FUNCTION_BLOCK FB_SFP_PPD_IO_LINK_ACYCLIC_DATA_V1_0_0
//-------------------------------------
VAR_INPUT

b_RELEASE								: BOOL;
i_READ_WRITE							: INT; 						// 1 = Read Index / 2 = Read All Parameter / 3 = Wright Index / 4 = Wright All Parameter
b_START									: BOOL;
s_NETID 								: STRING(23); 				// T_AmsNetId
i_IO_LINK_PORT_NR						: UINT;						// Port Number of IO-Link Master
w_INDEX 								: WORD			:= 16#00;
i_AREA_A								: INT;						// Parameter 66
i_AREA_B								: INT;						// Parameter 67
di_PISTON_STROKE : DINT;											// Parameter 68
di_FINGER_STROKE						: DINT;						// Parameter 177
ui_PREPOSITION_DELTA					: UINT;						// Parameter 178

END_VAR
//-------------------------------------
VAR_OUTPUT
	
    b_DONE											: BOOL;
    b_BUSY 											: BOOL;
    b_ERROR 										: BOOL;
	i_AREA_A_READ									: INT;	// Parameter 16#66
	i_AREA_B_READ									: INT;	// Parameter 16#67
	di_PISTON_STROKE_READ 	: DINT;	// Parameter 16#68
	di_FINGER_STROKE_READ							: DINT; // Parameter 16#177
	ui_PREPOSITION_DELTA_READ						: UINT; // Parameter 16#178

END_VAR
//-------------------------------------
VAR_STAT
	// Ab Hier soll alles Stat_Var sein
	
	Read_Write_Started	: BOOL; // Hilfsbit welches sich merkt, dass das Lesen und schreiben schon mal angestoßen wurde
	Index				: WORD;	// Index welcher über die Eingangsdaten eingelesen wird wird hier gespeichert
	Next_Parameter		: INT; // Welcher Parameter soll gelesen/geschrieben werden
	Next_Parameter_OLD	: INT; // Welcher Parameter wurde gelesen/geschrieben
	
// Struktur der Aktuell eingelesenen Parameter
	Parameter_Aktuell_i_Area_A									: INT; // 0x66 
	Parameter_Aktuell_i_Area_B									: INT; // 0x67
	Parameter_Aktuell_di_PISTON_STROKE	: DINT; // 0x68
	Parameter_Aktuell_di_Finger_Stroke							: DINT; // 0x177
	Parameter_Aktuell_di_Preposition_Delta						: UINT; // 0x178
	
	// Flanke zur Auswertung des Start Eingangs
	R_TRIG_instance_START	: R_TRIG;
	R_TRIG_instance_START_Q : BOOL;
	
	R_TRIG_WRREC_Error		: R_TRIG; // Triggerauswertung wenn beim Schreiben von Parametern etwas schiefgegangen ist
	R_TRIG_WRREC_Error_Q	: BOOL;
	
	
	Count_Write 		: INT; // Interner Hilfszähler
	Count_Write_Error 	: INT; // Interner schreib Fehlerzähler
	
	help_Valid_Done 	: BOOL; // Hilfsbit das Lesen oder Schreiben fertig sind
	help_Error 			: BOOL; // Hilfsbit Wenn ein Fehler auftritt

	// Struktur um Interne Error Bits auszuwerten 
	Error_struct_Error_Read_Write						: BOOL;
	Error_struct_Area_A									: BOOL;
	Error_struct_Area_B									: BOOL;
	Error_struct_PISTON_STROKE	: BOOL;
	Error_struct_Finger_Stroke							: BOOL;
	Error_struct_Preposition_Delta						: BOOL;
	
	Help_Index_Counter 									: DINT; // Bei Schritt 99 wird der letzte Index gesichert
		
	// Bausteine aus IO_Link Lib
	FB_IolRead				: FB_IolRead;
	FB_IolWrite				: FB_IolWrite;
		
	// Funktionsbausteine 
	FB_Parameter_Lesen_ADSREAD 		: ADSREAD;	// Funktionsbaustein zum Daten Azyklisch lesen 
	FB_Parameter_Schreiben_ADSWRITE	: ADSWRITE; // Funktionsbaustein zum Daten Azyklisch schreinen

	
	dw_Help_Storage_Copy	: DWORD;
	uint_Help_Storage_Copy	: UINT;
	dw_Help_Storage_Write	: DWORD;
	b_Help_Busy				: BOOL;
	
	// Zeit
	//FB_Time_Delay_Valid_Done : ton;

	t_Timeout : TIME := DEFAULT_ADS_TIMEOUT;
	 
	// ADSREAD Varriablen
	// OUTPUT	  
	  
	Length_DATA_WRITE	: UDINT;

	// Read Parameter 
		
	Help_last_round: BOOL;
	
	Help_Wartezeit: TON;
	Help_Wartezeit_Q : BOOL;
	Help_Wartezeit_time: TIME;
	
	Test_B_Trig_Start_Q: BOOL;
	temp_FB_IolWrite_bDone_Help: BOOL;
END_VAR	

//#################	
VAR	

END_VAR	  

//#################
VAR_TEMP 
	temp_FB_IolRead_bBusy		: BOOL;
	temp_FB_IolRead_bDone		: BOOL;
	temp_FB_IolRead_bError		: BOOL;
	temp_FB_IolRead_hresult		: DINT;
	temp_FB_IolRead_nAdsError	: UDINT;
	temp_FB_IolRead_nIolError	: UDINT;
	
	temp_FB_IolWrite_bBusy		: BOOL;
	temp_FB_IolWrite_bDone		: BOOL;
	temp_FB_IolWrite_bError		: BOOL;
	temp_FB_IolWrite_hresult	: DINT;
	temp_FB_IolWrite_nAdsError	: UDINT;
	temp_FB_IolWrite_nIolError	: UDINT;
		
END_VAR
//#################
VAR PERSISTENT
	
END_VAR



(*
	FUNCTION_BLOCK FB_ACYCLIC_COMMUNICATION
	TITLE = 'FB_Azyclic_Communication_SFP'
	VERSION : '1.0.0'
	AUTHOR  : 'SCHUNK'
	NAME    : 'FB_Azyclic_Communication_SFP'
	FAMILY  : 'SCHUNK'
	Projekt Nr.:
	=============================================================================
	 Schunk GmbH&Co.KG
	 (c)Copyright (2023) All Rights Reserved
	-----------------------------------------------------------------------------
	 Library:       Schunk
	 Tested with:   TwinCAT_3 Build 4024.47
	 Engineering:   TwinCAT 3 Build 4024.47
	 Restrictions:  XXX(OB types, etc.)
	 Requirements:  (hardware, technological package, memory needed, etc.)
	 Functionality: The Funktion Block communicates Azyclic with the Gripper to read and Write Data
	 
	 !!!!!!!!!!!!!!!!!!!!
	 !!!!! Atention !!!!!
	 !!!!!!!!!!!!!!!!!!!! 
	 Used Library of TwinCAT : TC2_EtherCAT V 3.3.15.0 (This library has to be installed) 
	 !!!!!!!!!!!!!!!!!!!!!!!!!!!!!!!!!!!!!!!!!!!!!!!!!!!!!!!!!!!!!!!!!!!!!!!!!!!!!!!!!!!!! 
	*************************************************************************
	Historie
	
	####################
	1.0.0
	Release Funktion Block
	
	
	*************************************************************************)
	    
	
(* MANUAL ENGLISH 
		    
    The block should have acyclic parameters, which can be changed for certain operator functions in order to make the application process safer or faster.
    
    input parameters:
    ==================
    
    b_RELEASE               :   TRUE = block is released for processing
    
    b_READ_WRITE            :    1 = the specified index parameter is read out and made available at the output parameters
                                 2 = all parameters available at the block are read and made available at the output parameters
                                 3 = the specified index parameter is written with the associated value
                                 4 = all parameters available on the block are written with the specified values
                        
    b_START                 :   Starts the write/read process.
    
    HW_IO                   :   Hardware address of the device can be found in the hardware parameterization
    
    dw_INDEX                :   Parameter address in hex format. The parameter must be specified if a single parameter is to be read or written. if all parameters are read or written, this parameter is not important because the block makes the parameter entries independently.
    
    i_AREA_A                :   66 The PPD shall provide the following parameter to parameterize the piston area of side A.
    
    i_AREA_B                :   67 The PPD shall provide the following parameter to parameterize the piston area of side B. 
    
    di_PISTON_STROKE        :   68 The PPD shall provide the following parameter to parameterize the piston stroke.  
    
    di_FINGER_STROKE        :   177 The PPD shall provide the following parameter to parameterize the the stroke per jaw.
    
    ui_PREPOSITION_DELTA    :   178 The PPD shall provide the following parameter to parameterize the the stroke between the workpiece window and the preposition.
        
    !!!!!!!!!!!!!!!!!!!!!!!!!!!!!!!!!!!!!!!!!!!!!!!!!!!!!!!!!!!!!!!!!!!!!!!!!!!!!!!!!!!!!!!!!!!!!!!!!!!!!!!!!!!!!!!!!!

    !!!!!!!!!!!!!!!!!!!!!!!!!!!!!!!!!!!!!!!!!!!!!!!!!!!!!!!!!!!!!!!!!!!!!!!!!!!!!!!!!!!!!!!!!!!!!!!!!!!!!!!!!!!!!!!!!!   
          
    output parameters:
    =================
    
    b_VALID_DONE                :   Feedback, job completed without errors
    
    b_BUSY                      :   Order is in progress
    
    b_ERROR                     :   Job completed, one or more parameters could not be read or written.
    
    i_AREA_A_READ               :   Value read the PPD shall provide the following parameter to parameterize the piston area of side A.
    
    i_AREA_B_READ               :   Value read the PPD shall provide the following parameter to parameterize the piston area of side B. 
    
    di_PISTON_STROKE_READ       :   Value read the PPD shall provide the following parameter to parameterize the piston stroke.
    
    di_FINGER_STROKE_READ       :   Value read the PPD shall provide the following parameter to parameterize the the stroke per jaw.
    
    ui_PREPOSITION_DELTA_READ   :   Value read the PPD shall provide the following parameter to parameterize the the stroke between the workpiece window and the preposition.
                   
    Caution:        If an error occurs after or during writing, the respective bit is set in the static data under "Error_struct" 
                    for which parameter the writing process could not be executed. 
                    The error message bits are retained until the block is triggered again via the "b_START" input parameter.
                
*************************************************************************)


// MANUAL GERMAN
    
(*************************************************************************
    Der Baustein soll azyklische Parameter, welche für bestimmte Funktionen von Operatoren geändert werden können um den Applikationsprozess sicherer oder schneller zu machen.
    
    Eingangsparameter:
    ==================
    
    b_RELEASE               :   TRUE = Baustein ist zur Bearbeitung freigegeben
    
    b_READ_WRITE            :   1 = der Angegebene Indexparameter wird ausgelesen und an den Ausgangsparametern zur Verfügung gestellt 
                                2 = alle am Baustein verfügbaren Parameter werden gelesen und an den Ausgangsparametern zur Vefügung gestellt
                                3 = der Angegebene Indexparameter wird mit dem zugehörigen Wert geschrieben
                                4 = alle am Baustein verfügbaren Parameter werden mit den angegebenen Werten beschrieben
                        
    b_START                 :   Startet den Schreib / Leseprozess.
    
    HW_IO                   :   Hardwareadresse des Gerätes aus der Hardwareparametrierung zu entnehmen
    
    dw_INDEX                :   Parameteradresse in Hex Format. Der Parameter muß angegeben werden wenn ein enzelner Parameter gelesen oder geschrieben werden soll. werden alle Parameter gelesen oder geschrieben ist dieser Parameter nicht von bedeutung, da der Baustein dei Parametereinträge selbständig vornimmt.
    
    i_AREA_A                :   66 Das PPD muss den folgenden Parameter zur Parametrisierung der Kolbenfläche der Seite A bereitstellen.
    
    i_AREA_B                :   67 Das PPD muss den folgenden Parameter zur Parametrisierung der Kolbenfläche der Seite B bereitstellen.
    
    di_PISTON_STROKE        :   68 Das PPD muss den folgenden Parameter zur Parametrierung des Kolbenhubs bereitstellen. 
    
    di_FINGER_STROKE        :   177 Das PPD muss den folgenden Parameter bereitstellen, um den Hub pro Backe zu parametrisieren.
    
    ui_PREPOSITION_DELTA    :   178 Das PPD muss den folgenden Parameter bereitstellen, um den Hub zwischen dem Werkstückfenster und der Vorposition zu parametrisieren.
    
    !!!!!!!!!!!!!!!!!!!!!!!!!!!!!!!!!!!!!!!!!!!!!!!!!!!!!!!!!!!!!!!!!!!!!!!!!!!!!!!!!!!!!!!!!!!!!!!!!!!!!!!!!!!!!!!
    Es ist darauf zu achten, dass beim SSCHreinen alle Parameter die richtigen Werte bei 
        Min_Position
        Max_Position
        Zero_Pos_Offset
    eingetragen sind, da es sonnst zu einer Störung oder falschen werten im Greifer kommen kann.
    
    Weitere Details zu den Parametern sind dem Handbuch des Gerätes zu entnehmen.
    !!!!!!!!!!!!!!!!!!!!!!!!!!!!!!!!!!!!!!!!!!!!!!!!!!!!!!!!!!!!!!!!!!!!!!!!!!!!!!!!!!!!!!!!!!!!!!!!!!!!!!!!!!!!!!!!   
    
    
    Ausgangsparameter:
    =================
    
    b_VALID_DONE                :   Rückmeldung, Auftrag beendet ohne Störungen
    
    b_BUSY                      :   Auftrag ist in Arbeit
    
    b_ERROR                     :   Auftrag abgeschlossen, ein oder mehrere Parameter konnten nicht gelesen oder geschrieben werden.
    
    i_AREA_A_READ               :   Der vom PPD gelesene Wert muss den folgenden Parameter bereitstellen, um die Kolbenfläche von Seite A zu parametrisieren.
    
    i_AREA_B_READ               :   Der vom PPD gelesene Wert muss den folgenden Parameter bereitstellen, um die Kolbenfläche von Seite B zu parametrisieren.
    
    di_PISTON_STROKE_READ       :   Der vom PPD gelesene Wert muss den folgenden Parameter zur Parametrierung des Kolbenhubs bereitstellen.
    
    di_FINGER_STROKE_READ       :   Der vom PPD gelesene Wert muss den folgenden Parameter bereitstellen, um den Hub pro Backe zu parametrisieren.
    
    ui_PREPOSITION_DELTA_READ   :   Der vom PPD gelesene Wert muss den folgenden Parameter bereitstellen, um den Hub zwischen dem Werkstückfenster und der Vorposition zu parametrisieren
    
    Achtung:    Trit nach dem schreiben ein Error auf, so wird in den Statischen Daten unter  "Error_struct" das jeweilige Bit,
                gesetzt bei welchem Parameter der Schreibvorgang nicht ausgeführt werden konnte.
                Die Störmeldebits bleiben so lange erhalten, bis ein erneutes anstoßen des Bausteins über den Eingangsparameter "b_START" erfolgt. 
                        
*************************************************************************)

// Release Prüfen
		// Release of the block is checked
	    // Freigabe des Bausteins wird geprüft 
	    	    
	    IF NOT b_RELEASE 
	    THEN
	        RETURN;
	    END_IF;
	    
//*******************************

// Start Eingang auswerten
	    // Start Trigger
	    // Start Flanke generieren
		
   IF NOT Read_Write_Started
        OR help_Error
    THEN
		R_TRIG_instance_START(CLK:= b_START, Q=> R_TRIG_instance_START_Q);
	END_IF;
		
//*******************************	
//Daten Ablöschen
// Reset Static Parameter
// Statische Parameter zurücksetzen
    IF R_TRIG_Instance_Start_Q
    THEN
		help_Valid_Done := FALSE;
        help_Error := FALSE;
        Error_struct_Error_Read_Write := 0;
        Error_struct_Area_A := FALSE;
        Error_struct_Area_B := FALSE;
        Error_struct_PISTON_STROKE := FALSE;
        Error_struct_Finger_Stroke := FALSE;
        Error_struct_Preposition_Delta := FALSE;
        Next_Parameter := 0;
    END_IF;
		
		
//*******************************
// Ablauf Lesen Schreiben	
	
	// Hilfsbit Lesen Schreiben ist gestartet
	
	    IF R_TRIG_Instance_Start_Q
	    THEN
	        Read_Write_Started := TRUE;
	    END_IF;
	//**********************   		
	
	// Index Wandeln von Word zu int
	Index := (w_INDEX);

	//**********************    
    IF Read_Write_Started 
		AND NOT help_Error
    THEN		    
	    CASE i_READ_WRITE OF
	            //******************************************
	         1: // Read One
	            // Read INDEX
	            // Lesen INDEX
	            
				Next_Parameter 	:= 0;	
				FB_IolRead.nIndex :=INDEX;
				FB_IolRead.bExecute := TRUE;
				//FB_Parameter_Lesen_ADSREAD.IDXOFFS := INDEX;
	            
	            //******************************************
	         2: // Read_All
	            // Read ALL
	            // Lesen ALLES
	            
	            IF R_TRIG_Instance_Start_Q
	                AND Next_Parameter = 0
	            THEN
	                Next_Parameter := 1;
					R_TRIG_Instance_Start_Q := FALSE;
	            END_IF;
	            
	            //************************    
					CASE Next_Parameter OF
							
						1: // i_AREA_A
							FB_IolRead.bExecute := TRUE; // b_Start_Read_Write := TRUE;
							FB_IolRead.nIndex := 66;
							;
						2: // i_AREA_B
							FB_IolRead.bExecute := TRUE; // b_Start_Read_Write := TRUE;
							FB_IolRead.nIndex := 67;
							;
						3: // di_PISTON_STROKE
							FB_IolRead.bExecute := TRUE; // b_Start_Read_Write := TRUE;
							FB_IolRead.nIndex := 68;
							;
						4: // di_FINGER_STROKE
							FB_IolRead.bExecute := TRUE; // b_Start_Read_Write := TRUE;
							FB_IolRead.nIndex := 177;
							;
						5: // ui_PREPOSITION_DELTA
							FB_IolRead.bExecute := TRUE; // b_Start_Read_Write := TRUE;
							FB_IolRead.nIndex := 178;
							;
						88: // Wait Step
                        	FB_IolRead.bExecute := FALSE;
                        	Next_Parameter := Next_Parameter_OLD + 1;
                        	Next_Parameter_OLD := 0
                        	;
                    	99: // Delete Step
                        	FB_IolRead.bExecute := FALSE;
                        	FB_IolRead.nIndex := 0;
                        	Next_Parameter := 0;
                        	Read_Write_Started := FALSE;
                        	;
						0: // Reset step
                        	FB_IolRead.bExecute := FALSE;
                        	FB_IolRead.nIndex := 0;
							;
					END_CASE;

	            //******************************************
	         3: // Write One
	            // Write INDEX
	            // Schreiben INDEX
	            
				Index := w_INDEX;	//?? Braucht man das noch weil es oben schon ist vor Case Anweisung
	
	            CASE Index OF

	                66: // i_AREA_A
	                    FB_IolWrite.bExecute := TRUE;
	                    MEMCPY(	destAddr	:= ADR(dw_Help_Storage_Write),
								srcAddr		:= ADR(i_AREA_A),
								n			:= 2)
								;
								
						dw_Help_Storage_Write := SHL(dw_Help_Storage_Write,16);
								
						dw_Help_Storage_Write := Host_To_Be32(in:= dw_Help_Storage_Write);		
						FB_IolWrite.nIndex := Index;
	                    Length_DATA_WRITE := 2;
	                    	                    
	                67: // i_AREA_B
	           			FB_IolWrite.bExecute := TRUE;
	                    MEMCPY(	destAddr	:= ADR(dw_Help_Storage_Write),
								srcAddr		:= ADR(i_AREA_B),
								n			:= 2)
								;
								
						dw_Help_Storage_Write := SHL(dw_Help_Storage_Write,16);
						
						dw_Help_Storage_Write := Host_To_Be32(in:= dw_Help_Storage_Write);
						FB_IolWrite.nIndex := Index;
	                    Length_DATA_WRITE := 2;

	                68: // di_PISTON_STROKE
						FB_IolWrite.bExecute := TRUE;
	                    MEMCPY(	destAddr	:= ADR(dw_Help_Storage_Write), 
								srcAddr		:= ADR(di_PISTON_STROKE),
								n			:= 4)
								;
						dw_Help_Storage_Write := Host_To_Be32(in:= dw_Help_Storage_Write);
				        FB_IolWrite.nIndex := Index;
	                    Length_DATA_WRITE := 4;
       
	                177: // di_FINGER_STROKE
						FB_IolWrite.bExecute := TRUE;
	                    MEMCPY(	destAddr	:= ADR(dw_Help_Storage_Write), 
								srcAddr		:= ADR(di_FINGER_STROKE),
								n			:= 4)
								;					
						dw_Help_Storage_Write := Host_To_Be32(in:= dw_Help_Storage_Write);
	                    FB_IolWrite.nIndex := Index;
	                    Length_DATA_WRITE := 4;

	                178: // ui_PREPOSITION_DELTA
						FB_IolWrite.bExecute := TRUE;
	                    MEMCPY(	destAddr	:= ADR(dw_Help_Storage_Write), 
								srcAddr		:= ADR(ui_PREPOSITION_DELTA),
								n			:= 4)
								;		
						dw_Help_Storage_Write := Host_To_Be32(in:= dw_Help_Storage_Write);
	                    FB_IolWrite.nIndex := Index;
	                    Length_DATA_WRITE := 4;
						
				ELSE
                        Help_Index_Counter := FB_IolWrite.nIndex;
                        FB_IolWrite.bExecute := FALSE;
                        FB_IolWrite.nIndex := 0;
                        Next_Parameter := 0;
                        Read_Write_Started := FALSE;
                        
                        help_Valid_Done := FALSE;
                        help_Error := TRUE;
						
	            END_CASE;
				
	            //******************************************
	         4: // Write_All
	            // Write ALL
	            // Schreiben ALLES
	            
	            IF R_TRIG_Instance_Start_Q AND
	                Next_Parameter = 0
	            THEN
	                Next_Parameter := 1;
					R_TRIG_Instance_Start_Q := FALSE; // Neu
	            END_IF;
	            //************************    
	            
				
				//IF FB_IolWrite.bExecute = FALSE 
					//AND FB_IolWrite.bBusy = FALSE
					//AND FB_IolWrite.bError = FALSE
					//AND b_ERROR = FALSE
					//THEN
				
					CASE Next_Parameter OF
							
						1: // i_AREA_A
							FB_IolWrite.bExecute := TRUE;
							FB_IolWrite.nIndex := 66;
														
							MEMCPY(	destAddr	:= ADR(dw_Help_Storage_Write),
									srcAddr		:= ADR(i_AREA_A),
									n			:= 2)
									;
									
							dw_Help_Storage_Write := SHL(dw_Help_Storage_Write,16);
							dw_Help_Storage_Write := Host_To_Be32(in:= dw_Help_Storage_Write);		
							Length_DATA_WRITE := 2;
						
						2: // i_AREA_B
							FB_IolWrite.bExecute := TRUE;
							FB_IolWrite.nIndex := 67;
							
							MEMCPY(	destAddr	:= ADR(dw_Help_Storage_Write), 
									srcAddr		:= ADR(i_AREA_B),
									n			:= 2)
									;
									
							dw_Help_Storage_Write := SHL(dw_Help_Storage_Write,16);		
							dw_Help_Storage_Write := Host_To_Be32(in:= dw_Help_Storage_Write);
							Length_DATA_WRITE := 2;
						
						3: // di_PISTON_STROKE
							FB_IolWrite.bExecute := TRUE;
							FB_IolWrite.nIndex := 68;
							
							MEMCPY(	destAddr	:= ADR(dw_Help_Storage_Write), 
									srcAddr		:= ADR(di_PISTON_STROKE),
									n			:= 4)
									;				
							dw_Help_Storage_Write := Host_To_Be32(in:= dw_Help_Storage_Write);
							Length_DATA_WRITE := 4;

						
						4: // di_FINGER_STROKE
							FB_IolWrite.bExecute := TRUE;
							FB_IolWrite.nIndex := 177;
						
							MEMCPY(	destAddr	:= ADR(dw_Help_Storage_Write), 
									srcAddr		:= ADR(di_FINGER_STROKE),
									n			:= 4)
									;
							dw_Help_Storage_Write := Host_To_Be32(in:= dw_Help_Storage_Write);
							Length_DATA_WRITE := 4;
						
						5: // ui_PREPOSITION_DELTA
							FB_IolWrite.bExecute := TRUE;
							FB_IolWrite.nIndex := 178;
							
							MEMCPY(	destAddr	:= ADR(dw_Help_Storage_Write), 
									srcAddr		:= ADR(ui_PREPOSITION_DELTA),
									n			:= 4)
									;
							dw_Help_Storage_Write := SHL(dw_Help_Storage_Write,16);
							dw_Help_Storage_Write := Host_To_Be32(in:= dw_Help_Storage_Write);
							Length_DATA_WRITE := 2;
														
						88: // Wait Step
                        	FB_IolWrite.bExecute := FALSE;
                        	Next_Parameter := Next_Parameter_OLD + 1;
                        	Next_Parameter_OLD := 0;
						
						99: // Last
                        	Help_Index_Counter := FB_IolWrite.nIndex;
                        	FB_IolWrite.bExecute := FALSE;
                        	FB_IolWrite.nIndex := 0;
                        	Next_Parameter := 0;
                        	Read_Write_Started := FALSE;
													
						END_CASE;
					
	    ELSE 
			RETURN; // Return von End Case #b_READ_WRITE
	    END_CASE;
	END_IF;
		
		
//######################################################################################################################
//######################################################################################################################
//######################################################################################################################	
//  Azyklisch lesen
	    // hier wird der Baustein angestoßen um einen Parameter zu schreiben
	    // Parameter Read Block
	    
	    IF i_READ_WRITE = 1 						// 1 = einen Parameter Lesen
	        OR i_READ_WRITE = 2						// 2 = alle Parameter Lesen
	        AND Next_Parameter <=99
	    THEN
	        
	        IF R_TRIG_Instance_Start_Q				// Lesen Starten
	        THEN
	            //FB_IolRead.bExecute := TRUE;
	            help_Valid_Done := FALSE;
	        END_IF;		
				
			FB_IolRead(
				bExecute	:= FB_IolRead.bExecute,    //b_Start_Read_Write, 
				sNetId		:= s_NETID, 
				nIolPort	:= i_IO_LINK_PORT_NR, 
				nIndex		:= FB_IolRead.nIndex,			// w_Gripper_Index_VAR, 
				nSubindex	:= 0, 
				pDSTBuf		:= ADR(DW_Help_Storage_Copy), //Pointer_Read_Index_1, //ADR(stat_grp_prehold_time),, 
				cbBufLen	:= SIZEOF(DW_Help_Storage_Copy),// Length_DATA_READ,//, 
				tTimeout	:= t_Timeout, 
				bBusy		=> temp_FB_IolRead_bBusy, 
				bDone		=> temp_FB_IolRead_bDone, 
				bError		=> temp_FB_IolRead_bError, 
				hresult		=> temp_FB_IolRead_hresult, 
				nAdsError	=> temp_FB_IolRead_nAdsError, 
				nIolError	=> temp_FB_IolRead_nIolError);

		END_IF;	      
  			
		//*************************************************
		// Daten in Statische Parameter schreiben 
		// Write Data into Static Parameter
		
	IF FB_IolRead.bBusy
    THEN
        FB_IolRead.bExecute := FALSE;
        help_Error := FALSE;
        //#Read_Write_Started := FALSE;
        
    ELSIF FB_IolRead.bError
    THEN
        help_Error := FB_IolRead.bError;
        FB_IolRead.bExecute := FALSE;
        //#Read_Write_Started := FALSE;
        Next_Parameter := 0;
        
    ELSIF FB_IolRead.bDone = TRUE
    THEN
        FB_IolRead.bExecute := FALSE;
        
        IF i_READ_WRITE = 1
        THEN
            help_Valid_Done := TRUE;
            help_Error := FALSE;
            
            Read_Write_Started := FALSE;
            
        ELSIF i_READ_WRITE = 2
            AND Next_Parameter < 6
        THEN
            //#Next_Parameter := #Next_Parameter + 1;
            IF Next_Parameter >= 5
            THEN
                help_Valid_Done := TRUE;
                help_Error := FALSE;
                
                Next_Parameter_OLD := Next_Parameter;
                Next_Parameter := 99;
            ELSE
                //END_IF;
                Next_Parameter_OLD := Next_Parameter;
                Next_Parameter := 88;
            END_IF;
            
        END_IF;
        
        // Kopieren aus dem Empfangsfach in die Ausgabedaten 
        CASE FB_IolRead.nIndex OF
            
			66: // i_AREA_A
				DW_Help_Storage_Copy := Host_To_Be32(in:= DW_Help_Storage_Copy);
				DW_Help_Storage_Copy := SHR(DW_Help_Storage_Copy,16);
				uint_Help_Storage_Copy := DWORD_TO_UINT(DW_Help_Storage_Copy);
				
				MEMCPY(	destAddr	:= ADR(Parameter_Aktuell_i_AREA_A), 
						srcAddr		:= ADR(uint_Help_Storage_Copy), 
						n			:= 4);
				DW_Help_Storage_Copy := 0;    
            						
			67: // i_AREA_B
				DW_Help_Storage_Copy := Host_To_Be32(in:= DW_Help_Storage_Copy);
				DW_Help_Storage_Copy := SHR(DW_Help_Storage_Copy,16);
				uint_Help_Storage_Copy := DWORD_TO_UINT(DW_Help_Storage_Copy);
				
				MEMCPY(	destAddr	:= ADR(Parameter_Aktuell_i_Area_B), 
						srcAddr		:= ADR(DW_Help_Storage_Copy), 
						n			:= 4);
				DW_Help_Storage_Copy := 0;

            68: // di_PISTON_STROKE
				DW_Help_Storage_Copy := Host_To_Be32(in:= DW_Help_Storage_Copy);
				
				MEMCPY(	destAddr	:= ADR(Parameter_Aktuell_di_PISTON_STROKE), 
						srcAddr		:= ADR(DW_Help_Storage_Copy), 
						n			:= 4);
				DW_Help_Storage_Copy := 0;
		
            177: // di_FINGER_STROKE
				DW_Help_Storage_Copy := Host_To_Be32(in:= DW_Help_Storage_Copy);
				
				MEMCPY(	destAddr	:= ADR(Parameter_Aktuell_di_Finger_Stroke), 
						srcAddr		:= ADR(DW_Help_Storage_Copy), 
						n			:= 4);
				DW_Help_Storage_Copy := 0;
                 
			178: // ui_PREPOSITION_DELTA
				DW_Help_Storage_Copy := Host_To_Be32(in:= DW_Help_Storage_Copy);
				DW_Help_Storage_Copy := SHR(DW_Help_Storage_Copy,16);
				uint_Help_Storage_Copy := DWORD_TO_UINT(DW_Help_Storage_Copy);
				
				MEMCPY(	destAddr	:= ADR(Parameter_Aktuell_di_Preposition_Delta), 
						srcAddr		:= ADR(DW_Help_Storage_Copy), 
						n			:= 2);
				DW_Help_Storage_Copy := 0;
                        
            ELSE
                Help_Index_Counter := FB_IolRead.nIndex;
                FB_IolRead.bExecute := FALSE;
                FB_IolRead.nIndex:= 0;
                Next_Parameter := 0;
                Read_Write_Started := FALSE;
                
                help_Valid_Done := FALSE;
                help_Error := TRUE;
                 
        END_CASE;
    END_IF;

//#############################################################################################	
// Azyklisch Schreiben 
		
	IF i_READ_WRITE = 3
        OR i_READ_WRITE = 4
    THEN
	
		//IF R_TRIG_Start.Q
		//THEN
          //  b_VALID_DONE := FALSE;
		//END_IF;	
		
		FB_IolWrite(
			bExecute	:= FB_IolWrite.bExecute, 
			sNetId		:= s_NETID, 
			nIolPort	:= i_IO_LINK_PORT_NR, 
			nIndex		:= FB_IolWrite.nIndex, 
			nSubindex	:= , 
			pSRCBuf		:= ADR(dw_Help_Storage_Write), 
			cbBufLen	:= Length_DATA_WRITE,	//2, //SIZEOF(Var_test_Wright), , 
			tTimeout	:= t_Timeout, 
			bBusy		=> temp_FB_IolWrite_bBusy, 
			bDone		=> temp_FB_IolWrite_bDone, 
			bError		=> temp_FB_IolWrite_bError, 
			hresult		=> temp_FB_IolWrite_hresult, 
			nAdsError	=> temp_FB_IolWrite_nAdsError, 
			nIolError	=> temp_FB_IolWrite_nIolError);

// Auswertung Error Bit von Baustein um den Fehler zu bestimmen			
        R_TRIG_WRREC_Error(CLK := FB_IolWrite.bError,
                            Q => R_TRIG_WRREC_Error_Q);

        IF R_TRIG_WRREC_Error_Q
        THEN
            Count_Write_Error := Count_Write_Error + 1;
            help_Error := TRUE;
            Read_Write_Started := FALSE;
            
            CASE FB_IolWrite.nIndex OF
                    
                66: // ui_GRIP_PREHOLD_TIME
                    Error_struct_Area_A := TRUE;
                    
                67: // r_Margin for workpiece detection
                    Error_struct_Area_B := TRUE;
                    
                68: // r_Gripping pre-position delta
                    Error_struct_PISTON_STROKE := TRUE;
                    
                177: // r_WP_RELEASE_DELTA
                    Error_struct_Finger_Stroke := TRUE;
                    
                178: // r_WP_LOST_DISTANCE
                    Error_struct_Preposition_Delta := TRUE;
                                                  
            END_CASE;
        END_IF;

        // Reset Bits when Error or done         
        
        IF i_READ_WRITE = 3
            OR i_READ_WRITE = 4
        THEN
//#########################            
            IF FB_IolWrite.bDone		// Schreiben fertig
			THEN
				temp_FB_IolWrite_bDone_Help:= TRUE;
			END_IF;	

			Help_Wartezeit(IN:= temp_FB_IolWrite_bDone_Help,
							PT:= T#5S, 
							Q=> Help_Wartezeit_Q, 
							ET=> Help_Wartezeit_time);			
			
			IF Help_Wartezeit_Q
//########################
			THEN
                FB_IolWrite.bExecute := FALSE;
				temp_FB_IolWrite_bDone_Help := FALSE;
                // Hilfszähler
                Count_Write := Count_Write + 1;
                
                IF i_READ_WRITE = 3
                THEN
                    help_Valid_Done := TRUE;
                    help_Error := FALSE;
                    Read_Write_Started := FALSE;
                    FB_IolWrite.bExecute := FALSE;
                    
                ELSIF i_READ_WRITE = 4
                THEN
                    IF Next_Parameter >= 5
                    THEN
                        help_Valid_Done := TRUE;
                        help_Error := FALSE;
						                        
                        Next_Parameter_OLD := Next_Parameter;
                        Next_Parameter := 99;
                    ELSE
                        //END_IF;
                        Next_Parameter_OLD := Next_Parameter;
                        Next_Parameter := 88;
                    END_IF;
                END_IF;
            END_IF;
            
            IF FB_IolWrite.bError
            THEN
                
                FB_IolWrite.bExecute := FALSE;
                
                IF i_READ_WRITE = 4
                THEN
                    Next_Parameter_OLD := Next_Parameter;
                    Next_Parameter := 88;
                END_IF;
            END_IF;
        END_IF;
    END_IF;
    

// Ausgangsparameter kopieren
       
    IF Error_struct_Area_A OR
       Error_struct_Area_B OR
       Error_struct_PISTON_STROKE OR
       Error_struct_Finger_Stroke OR
       Error_struct_Preposition_Delta
    THEN
       help_Error := TRUE;
       
    END_IF;
    
    
    b_BUSY := FB_Iolread.bBusy OR FB_IolWrite.bBusy OR temp_FB_IolWrite_bDone_Help;
    b_Done := help_Valid_Done;
    b_ERROR := help_Error;
    
    i_AREA_A_READ									:= Parameter_Aktuell_i_Area_A;
    i_AREA_B_READ									:= Parameter_Aktuell_i_Area_B;
    di_PISTON_STROKE_READ							:= Parameter_Aktuell_di_PISTON_STROKE;
    di_FINGER_STROKE_READ							:= Parameter_Aktuell_di_Finger_Stroke;
    ui_PREPOSITION_DELTA_READ						:= Parameter_Aktuell_di_Preposition_Delta;

END_FUNCTION_BLOCK
